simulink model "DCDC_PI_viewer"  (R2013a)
settings: Solver=ode45  StartTime=0.0  StopTime=8e-3  RelTol=1e-3
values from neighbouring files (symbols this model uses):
  Do = 0.4166    [DCDCConverter.m]
undefined symbols (not defined in the file or in its folder): plecs
libraries: simulink x1

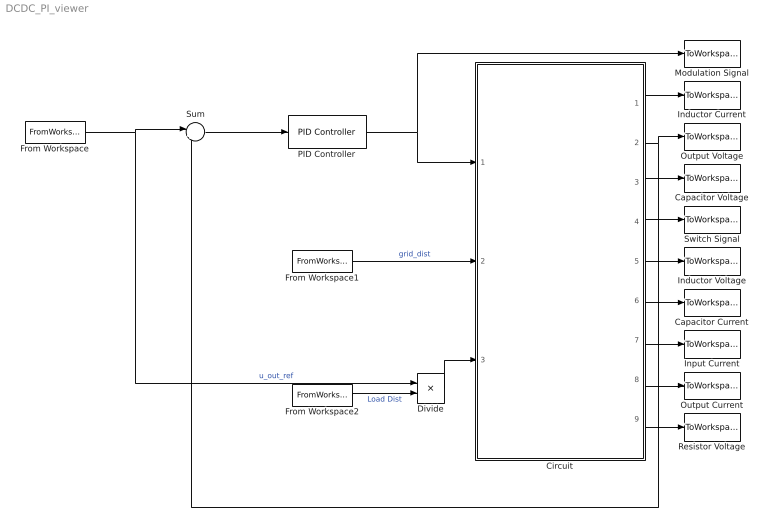
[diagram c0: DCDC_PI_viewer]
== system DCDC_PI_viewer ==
  Capacitor Current : ToWorkspace  VariableName=i_R_PI  SampleTime=-1  SaveFormat=Timeseries
  Capacitor Voltage : ToWorkspace  VariableName=u_C_PIPlecs  SampleTime=-1  SaveFormat=Timeseries
  Circuit : Subsystem  LoadFcn=plecs('sl', 200);  InitFcn=plecs('sl', 214);  StartFcn=plecs('sl', 208);  StopFcn=plecs('sl', 209);
  Divide : Product  Inputs=*/
  From Workspace : FromWorkspace  VariableName=[t, U_out_ref_PL]  SampleTime=0
  From Workspace1 : FromWorkspace  VariableName=[t, Grid_Dist_PL]  SampleTime=0
  From Workspace2 : FromWorkspace  VariableName=[t, Load_Dist_PL]  SampleTime=0
  Inductor Current : ToWorkspace  VariableName=i_L_PIPlecs  SampleTime=-1  SaveFormat=Timeseries
  Inductor Voltage : ToWorkspace  VariableName=u_L_PI  SampleTime=-1  SaveFormat=Timeseries
  Input Current : ToWorkspace  VariableName=i_IN_PIPlecs  SampleTime=-1  SaveFormat=Timeseries
  Modulation Signal : ToWorkspace  VariableName=m_PI  SampleTime=-1  SaveFormat=Timeseries
  Output Current : ToWorkspace  VariableName=i_OUT_PIPlecs  SampleTime=-1  SaveFormat=Timeseries
  Output Voltage : ToWorkspace  VariableName=U_out_PIPlecs  SampleTime=-1  SaveFormat=Timeseries
  PID Controller : simulink/Continuous/PID Controller  Controller=PID  TimeDomain=Continuous-time  SampleTime=1  IntegratorMethod=Forward Euler  FilterMethod=Forward Euler  Form=Parallel  P=.4/Do  I=2*pi*641*.4/Do  D=0  N=100  InitialConditionSource=internal  InitialConditionForIntegrator=0  InitialConditionForFilter=0  ExternalReset=none  LimitOutput=on  UpperSaturationLimit=1  LowerSaturationLimit=0  LinearizeAsGain=on  AntiWindupMode=back-calculation  Kb=1  TrackingMode=off  Kt=1  PParamMin=[]  PParamMax=[]  IParamMin=[]  IParamMax=[]  DParamMin=[]  DParamMax=[]  NParamMin=[]  NParamMax=[]  KbParamMin=[]  KbParamMax=[]  KtParamMin=[]  KtParamMax=[]  POutMin=[]  POutMax=[]  IOutMin=[]  IOutMax=[]  DOutMin=[]  DOutMax=[]  NOutMin=[]  NOutMax=[]  KbOutMin=[]  KbOutMax=[]  KtOutMin=[]  KtOutMax=[]  IntegratorOutMin=[]  IntegratorOutMax=[]  FilterOutMin=[]  FilterOutMax=[]  SumOutMin=[]  SumOutMax=[]  SumI1OutMin=[]  SumI1OutMax=[]  SumI2OutMin=[]  SumI2OutMax=[]  SumI3OutMin=[]  SumI3OutMax=[]  SumDOutMin=[]  SumDOutMax=[]  SaturationOutMin=[]  SaturationOutMax=[]  IntegratorContinuousStateAttributes=''  IntegratorStateMustResolveToSignalObject=off  IntegratorRTWStateStorageClass=Auto  FilterContinuousStateAttributes=''  FilterStateMustResolveToSignalObject=off  FilterRTWStateStorageClass=Auto
  Resistor Voltage : ToWorkspace  VariableName=u_R_PI  SampleTime=-1  SaveFormat=Timeseries
  Sum : Sum  Inputs=|+-
  Switch Signal : ToWorkspace  VariableName=d_PLECS  SampleTime=-1  SaveFormat=Timeseries
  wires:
  PID Controller/1 -> Modulation Signal/1, Circuit/1(Mod Signal)
  From Workspace1/1 -> Circuit/2(Grid Voltage)  "grid_dist"
  Sum/1 -> PID Controller/1
  From Workspace/1 -> Divide/1, Sum/1  "u_out_ref"
  Circuit/1(i L) -> Inductor Current/1
  Circuit/2(U out) -> Sum/2, Output Voltage/1
  Circuit/3(u C) -> Capacitor Voltage/1
  Circuit/4(d Plecs) -> Switch Signal/1
  Circuit/5(u L) -> Inductor Voltage/1
  Circuit/6(i R) -> Capacitor Current/1
  Circuit/7(i IN) -> Input Current/1
  Circuit/8(i OUT) -> Output Current/1
  Circuit/9(u R) -> Resistor Voltage/1
  From Workspace2/1 -> Divide/2  "Load Dist"
  Divide/1 -> Circuit/3(Load Resistance)

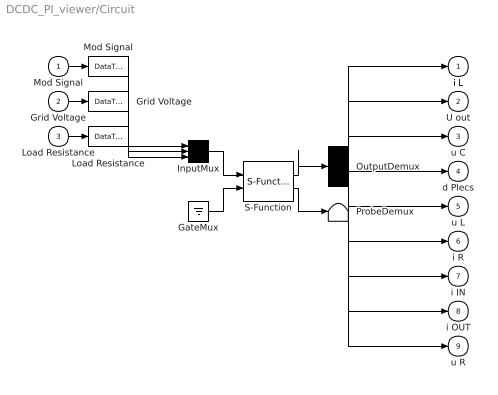
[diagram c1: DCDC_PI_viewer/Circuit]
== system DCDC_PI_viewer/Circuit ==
  Mod Signal : Inport  PortDimensions=1
  Grid Voltage : Inport  Port=2  PortDimensions=1
  Load Resistance : Inport  Port=3  PortDimensions=1
  " GateMux " : Ground
  " Grid Voltage " : DataTypeConversion
  " InputMux " : Mux  Inputs=[ 1 1 1 ]
  " Load Resistance " : DataTypeConversion
  " Mod Signal " : DataTypeConversion
  " OutputDemux " : Demux  Outputs=[ 1 1 1 1 1 1 1 1 1 ]
  " ProbeDemux " : Terminator
  " S-Function " : S-Function  FunctionName=plecs  EnableBusSupport=off
  i L : Outport  PortDimensions=1
  U out : Outport  Port=2  PortDimensions=1
  u C : Outport  Port=3  PortDimensions=1
  d Plecs : Outport  Port=4  PortDimensions=1
  u L : Outport  Port=5  PortDimensions=1
  i R : Outport  Port=6  PortDimensions=1
  i IN : Outport  Port=7  PortDimensions=1
  i OUT : Outport  Port=8  PortDimensions=1
  u R : Outport  Port=9  PortDimensions=1
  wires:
  " S-Function "/1 -> " OutputDemux "/1
  " InputMux "/1 -> " S-Function "/1
  " GateMux "/1 -> " S-Function "/2
  " S-Function "/2 -> " ProbeDemux "/1
  Mod Signal/1 -> " Mod Signal "/1
  " Mod Signal "/1 -> " InputMux "/1
  Grid Voltage/1 -> " Grid Voltage "/1
  " Grid Voltage "/1 -> " InputMux "/2
  Load Resistance/1 -> " Load Resistance "/1
  " Load Resistance "/1 -> " InputMux "/3
  " OutputDemux "/1 -> i L/1
  " OutputDemux "/2 -> U out/1
  " OutputDemux "/3 -> u C/1
  " OutputDemux "/4 -> d Plecs/1
  " OutputDemux "/5 -> u L/1
  " OutputDemux "/6 -> i R/1
  " OutputDemux "/7 -> i IN/1
  " OutputDemux "/8 -> i OUT/1
  " OutputDemux "/9 -> u R/1
